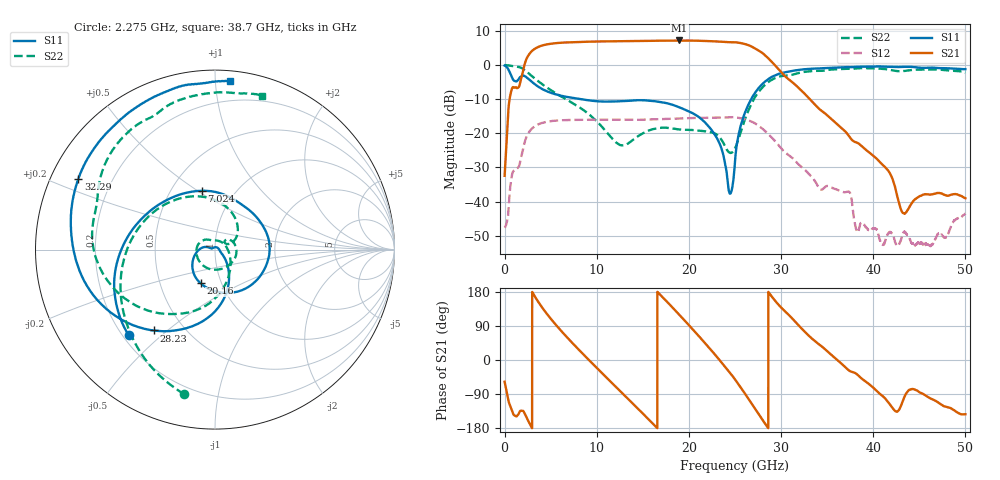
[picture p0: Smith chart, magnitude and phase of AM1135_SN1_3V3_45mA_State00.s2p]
!Agilent Technologies,E8364B,MY43040894,A.07.50.67
!Agilent E8364B: A.07.50.67
!Date: Monday, November 15, 2021 11:12:15
!Correction: S11(Full 2 Port(1,2))
!S21(Full 2 Port(1,2))
!S12(Full 2 Port(1,2))
!S22(Full 2 Port(1,2))
!S2P File: Measurements: S11, S21, S12, S22:
# Hz S  dB  R 50
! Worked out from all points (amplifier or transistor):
!   6401 points, 10 MHz to 50 GHz, reference 50 ohm
!   highest |S21| = 7.2 dB at 18.97 GHz (marker M1)
!   |S21| within 3 dB of that: 3.008 GHz to 27.61 GHz (24.6 GHz wide, 161 % of centre)
!   unconditionally stable (mu >= 1): 40.82 MHz to end of sweep
!   at 8.336 GHz: K = 1.42, MAG = 7.6 dB, |S12| = -16.0 dB
!   at 25 GHz: K = 1.53, MAG = 6.7 dB, |S12| = -15.3 dB
!   at 50 GHz: K = 666.83, MAG = -29.0 dB, |S12| = -43.5 dB
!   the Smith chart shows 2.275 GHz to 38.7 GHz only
!   S11 on the Smith chart (normalised r, x): 2.275 GHz: 0.22, -0.40; 7.024 GHz: 0.70, +0.52; 20.16 GHz: 0.80, -0.31; 28.23 GHz: 0.34, -0.45; 32.29 GHz: 0.08, +0.24; 38.7 GHz: 0.07, +1.09
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1e7  -0.18 -10.5  -32.44 -57.3  -47.62 -52.3  -0.01 -4.8
6.661188e8  -2.70 -58.8  -8.37 -124.1  -34.74 105.4  -0.24 -29.1
2.275172e9  -3.38 -135.1  1.02 -145.3  -21.81 57.7  -1.69 -102.1
3.860792e9  -6.70 163.1  5.49 146.2  -17.16 -14.0  -5.20 -162.9
5.391736e9  -8.48 129.9  6.33 97.9  -16.33 -61.4  -8.02 147.1
7.024222e9  -9.47 102.7  6.63 53.6  -16.10 -103.5  -10.58 99.9
8.34427e9  -10.03 84.5  6.76 20.1  -16.04 -134.4  -12.79 67.1
1.031263e10  -10.68 61.1  6.88 -28.2  -16.03 -178.8  -17.34 29.5
1.268715e10  -10.62 34.4  6.95 -85.5  -16.06 129.4  -23.52 32.6
1.447586e10  -10.32 8.5  7.00 -128.5  -16.05 90.9  -20.87 38.4
1.667854e10  -10.74 -32.5  7.09 177.6  -15.91 42.8  -18.49 -0.6
1.896715e10  -12.40 -83.6  7.17 119.4  -15.67 -9.2  -18.88 -65.6
2.016222e10  -13.80 -113.2  7.14 87.8  -15.55 -37.6  -19.02 -106.2
2.281013e10  -20.35 -175.8  6.91 14.9  -15.42 -104.5  -20.08 165.6
2.5005e10  -28.34 -27.0  6.65 -51.2  -15.30 -167.6  -24.40 28.7
2.637972e10  -12.07 -75.4  5.87 -99.4  -16.13 146.4  -13.84 -73.7
2.823092e10  -4.96 -127.2  2.92 -166.7  -19.26 81.7  -5.89 -138.3
3.22926e10  -1.33 152.5  -7.70 81.6  -29.97 -17.9  -2.14 140.6
3.333927e10  -1.11 138.8  -10.63 56.8  -32.81 -39.6  -1.78 126.3
3.869757e10  -0.52 84.8  -23.63 -47.9  -46.13 -113.4  -0.94 72.9
4.167354e10  -0.55 57.0  -31.11 -112.6  -49.17 -108.6  -1.36 44.0
5e10  -1.23 -63.4  -39.01 -143.0  -43.54 -106.5  -2.25 -68.3
